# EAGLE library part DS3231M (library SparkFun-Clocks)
DS3231M Real Time Clock Accuracy +/-5ppm. Battery Backup. 2.3V to 5.5V. Datasheet SparkFun Products CryptoCape (DEV-12773) SparkFun CryptoShield (DEV-13183)
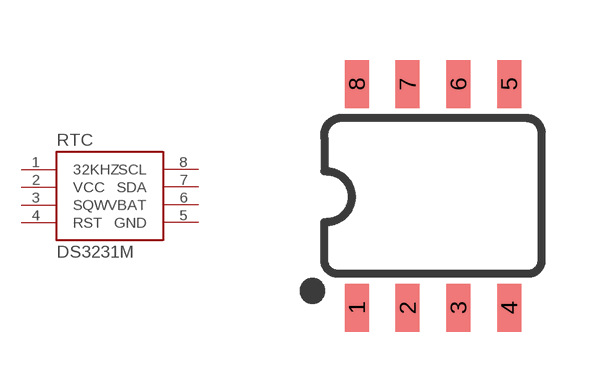
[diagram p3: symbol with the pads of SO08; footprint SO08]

Designator prefix RTC

## DS3231M (PROD_ID: IC-11985)  [SO08]
1  32KHZ  out
2  VCC  pwr
3  SQW  out
4  RST
5  GND  pwr
6  VBAT  pwr
7  SDA
8  SCL

## Footprint SO08 (pad centres in mm)
SOIC, 0.15 inch width
smd 0.6 x 1.2: 1 -1.905,-2.8; 2 -0.635,-2.8; 3 0.635,-2.8; 4 1.905,-2.8; 5 1.905,2.8; 6 0.635,2.8; 7 -0.635,2.8; 8 -1.905,2.8

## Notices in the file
Licensing: Creative Commons ShareAlike 4.0 International - https://creativecommons.org/licenses/by-sa/4.0
